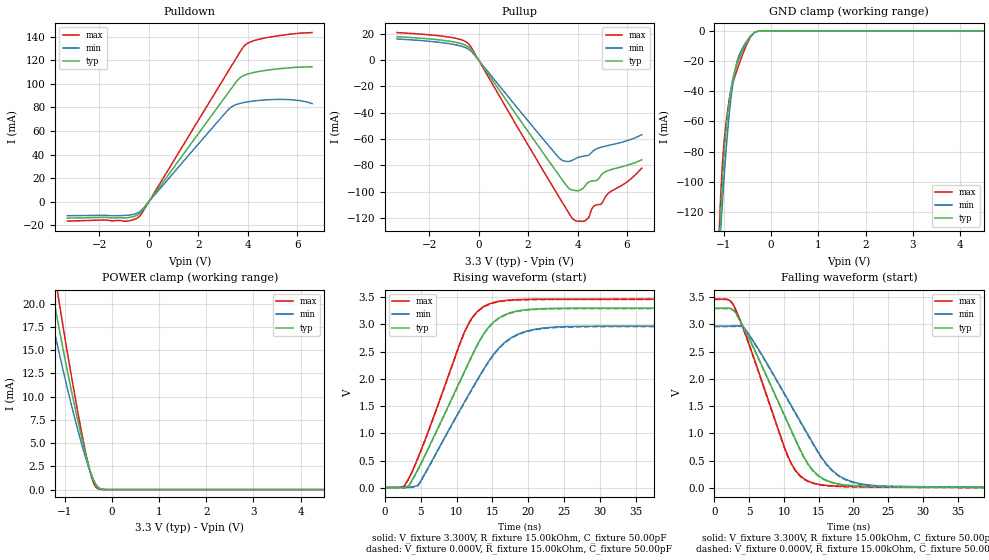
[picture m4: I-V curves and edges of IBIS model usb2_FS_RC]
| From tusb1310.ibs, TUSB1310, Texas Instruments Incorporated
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|   USB 2.0 Fast Speed mode, for DM pin 6MHz
[Model]   usb2_FS_RC
Model_type   I/O
Polarity   Non-Inverting
Enable   Active-High
Vmeas = 1.54
Vref = 0
Rref = 15000
Cref = 50pF
Vinl = 0.8V
Vinh = 2.0V
|   typ   min   max
|   (nom PVT)   (Fast PVT)   (slow PVT)
C_comp   9.0376pF   8.9385pF   9.1512pF
[Voltage Range]   3.3   2.97   3.465
[Temperature Range]   27   105   -40
[Pullup Reference]   3.3   2.97   3.465
[Pulldown Reference]   -0   -0   -0
[Power Clamp Reference]   3.3   2.97   3.465
[GND Clamp Reference]   -0   -0   -0
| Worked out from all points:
|   slope of the pulldown table from 0 to 0.495 V, typ, clamps not added: 34.6 ohm
|   slope of the pullup table from 0 to 0.495 V, typ, clamps not added: 36.8 ohm
|   GND clamp passes 1 mA (typ) near -0.35 V on its own axis
|   POWER clamp passes 1 mA (typ) near -0.39 V on its own axis
|   falling waveform, V_fixture 3.300V, R_fixture 15.00kOhm, C_fixture 50.00pF: 20-80 % time 7.09ns typ, 8.08ns min, 5.62ns max; typ from 3.3 V to 0.008 V
|   rising waveform, V_fixture 3.300V, R_fixture 15.00kOhm, C_fixture 50.00pF: 20-80 % time 7.12ns typ, 7.76ns min, 5.77ns max; typ from 0.008 V to 3.3 V
|   rising waveform, V_fixture 0.000V, R_fixture 15.00kOhm, C_fixture 50.00pF: 20-80 % time 7.12ns typ, 7.77ns min, 5.77ns max; typ from 0 V to 3.29 V
|   falling waveform, V_fixture 0.000V, R_fixture 15.00kOhm, C_fixture 50.00pF: 20-80 % time 7.08ns typ, 8.07ns min, 5.61ns max; typ from 3.29 V to 0 V
[Pulldown]
|   Voltage   I(typ)   I(min)   I(max)
-3.3V     -13.97mA   -11.94mA   -16.5mA
-1.865V   -13.31mA   -11.55mA   -15.58mA
-948.8mV  -13.78mA   -11.64mA   -16.64mA
-429mV    -11.05mA   -9.328mA   -13.36mA
-255.8mV  -7.37mA    -6.247mA   -8.827mA
3.234V    93.1mA     78.54mA    111.5mA
3.61V     103.6mA    82.92mA    124.4mA
3.858V    107.2mA    84.17mA    132.2mA
4.15V     109.1mA    85.16mA    135.8mA
4.714V    111.3mA    86.32mA    138.9mA
5.798V    113.7mA    86.37mA    142.3mA
6.6V      114.4mA    83.14mA    143.4mA
[GND Clamp]
|   Voltage   I(typ)   I(min)   I(max)
-3.3V     -2.986A    -2.594A    -3.408A
-1.102V   -142.8mA   -148.5mA   -133.6mA
-1.068V   -120.4mA   -130.9mA   -108.6mA
-1.053V   -111.5mA   -123.5mA   -99.43mA
-1.028V   -97.72mA   -111.6mA   -86.34mA
-948.8mV  -63.66mA   -76.9mA    -59.29mA
-874.5mV  -43.76mA   -51.14mA   -43.02mA
-795.3mV  -29.32mA   -31.84mA   -32.77mA
-676.5mV  -18.29mA   -15.93mA   -21.75mA
-458.7mV  -4.679mA   -4.168mA   -5.163mA
-349.8mV  -954.6uA   -1.019mA   -868.7uA
6.6V      27.44uA    21.44uA    34.47uA
[Pullup]
|   Voltage   I(typ)   I(min)   I(max)
-3.3V     17.86mA    16.11mA    20.95mA
-1.162V   14.34mA    12.44mA    17.42mA
-374.6mV  9.504mA    7.922mA    11.72mA
3.224V    -86.72mA   -73.66mA   -103.1mA
3.625V    -96.87mA   -77.02mA   -115.4mA
3.863V    -98.94mA   -75.34mA   -121.4mA
4.303V    -95.54mA   -72.68mA   -122mA
4.452V    -92.62mA   -72.08mA   -119.5mA
4.655V    -91.65mA   -68.64mA   -111mA
4.962V    -87.23mA   -66.09mA   -109.1mA
5.14V     -84.63mA   -65.26mA   -103.4mA
6.6V      -75.66mA   -56.61mA   -82.01mA
[POWER Clamp]
|   Voltage   I(typ)   I(min)   I(max)
-3.3V     96.11mA    80.39mA    114.3mA
-1.409V   25.5mA     21.48mA    30.05mA
-1.315V   22.86mA    19.29mA    26.86mA
-1.246V   20.93mA    17.7mA     24.52mA
-1.127V   17.68mA    15mA       20.59mA
-854.7mV  10.64mA    9.089mA    12.22mA
-567.6mV  4.132mA    3.664mA    4.338mA
-419.1mV  1.439mA    1.425mA    1.205mA
-359.7mV  684.8uA    768.2uA    455.6uA
-290.4mV  187uA      273.4uA    86.97uA
0V        0A         0A         0A
6.6V      0A         0A         0A
[Ramp]
R_load = 15.00kOhm
|   typ   min   max
dV/dt_r   1.975V/7.118ns   1.776V/7.768ns   2.074V/5.764ns
dV/dt_f   1.975V/7.089ns   1.777V/8.081ns   2.074V/5.614ns
[Falling Waveform]
V_fixture = 3.300V
V_fixture_min = 2.970V
V_fixture_max = 3.465V
R_fixture = 15.00kOhm
C_fixture = 50.00pF
|   Time   V(typ)   V(min)   V(max)
0s        3.299V     2.969V     3.464V
2.4ns     3.286V     2.97V      3.419V
4.2ns     2.947V     2.947V     2.907V
10.69ns   1.157V     1.59V      545mV
12.14ns   753.6mV    1.267V     246.5mV
14.07ns   335.9mV    840.6mV    94.42mV
15.85ns   154.3mV    481.3mV    48.71mV
17.64ns   77.37mV    248.2mV    32.68mV
22.25ns   29.92mV    52.16mV    21.45mV
83.29ns   7.582mV    8.019mV    6.667mV
[Rising Waveform]
V_fixture = 3.300V
V_fixture_min = 2.970V
V_fixture_max = 3.465V
R_fixture = 15.00kOhm
C_fixture = 50.00pF
|   Time   V(typ)   V(min)   V(max)
0s        7.582mV    8.019mV    6.667mV
2.63ns    14.86mV    8.107mV    23.09mV
3.35ns    42.86mV    10.65mV    176.9mV
4.68ns    354.6mV    57.1mV     571.4mV
11.34ns   2.202V     1.63V      2.927V
12.88ns   2.621V     1.981V     3.234V
14.9ns    3.01V      2.403V     3.391V
18.36ns   3.243V     2.808V     3.454V
23.8ns    3.294V     2.952V     3.463V
83.29ns   3.299V     2.969V     3.464V
[Rising Waveform]
V_fixture = 0.000V
V_fixture_min = 0.000V
V_fixture_max = 0.000V
R_fixture = 15.00kOhm
C_fixture = 50.00pF
|   Time   V(typ)   V(min)   V(max)
0s        3.197uV    8.923uV    4.349uV
2.63ns    7.278mV    96.94uV    16.39mV
3.36ns    36.84mV    2.771mV    171.8mV
4.68ns    345.4mV    48.95mV    562.8mV
11.35ns   2.193V     1.621V     2.921V
12.89ns   2.613V     1.97V      3.227V
14.91ns   3.001V     2.393V     3.384V
18.18ns   3.229V     2.786V     3.446V
23.01ns   3.284V     2.936V     3.456V
83.29ns   3.291V     2.961V     3.457V
[Falling Waveform]
V_fixture = 0.000V
V_fixture_min = 0.000V
V_fixture_max = 0.000V
R_fixture = 15.00kOhm
C_fixture = 50.00pF
|   Time   V(typ)   V(min)   V(max)
0s        3.291V     2.961V     3.457V
2.4ns     3.278V     2.961V     3.412V
4.2ns     2.937V     2.938V     2.898V
10.67ns   1.15V      1.581V     540.7mV
12.12ns   746.6mV    1.258V     240.7mV
14.05ns   328.3mV    831mV      87.96mV
15.83ns   146.5mV    471.7mV    42.08mV
17.61ns   69.9mV     239.9mV    26.07mV
22.23ns   22.29mV    43.83mV    14.8mV
83.29ns   3.197uV    8.923uV    4.349uV
